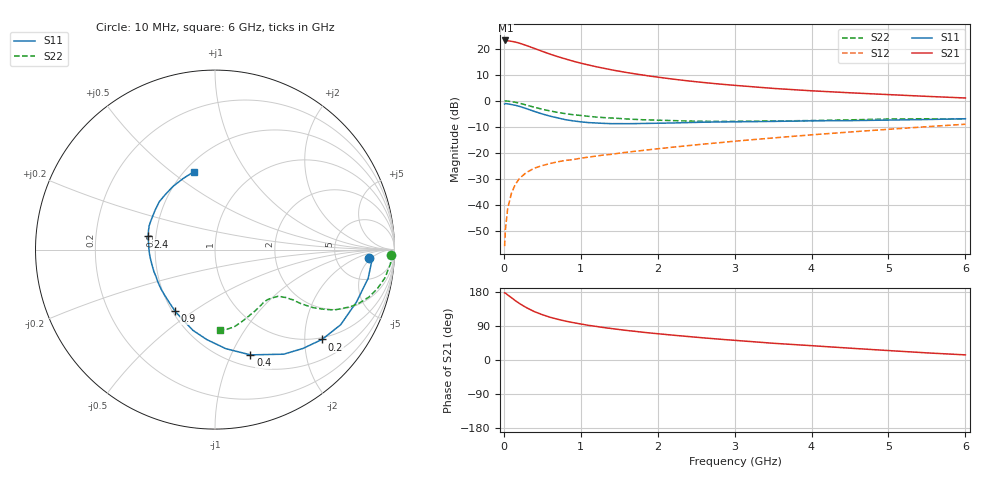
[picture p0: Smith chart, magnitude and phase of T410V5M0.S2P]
! Infineon Technologies  Discrete & RF Semiconductors
! BFR182T
! Si NPN RF Bipolar Junction Transistor in SC75
! VCE = 10 V  IC = 5 mA
! Common Emitter S-Parameters:  October  1999
# GHz  S  MA  R  50
!  f  S11  S21  S12  S22
! GHz  MAG  ANG  MAG  ANG  MAG  ANG  MAG  ANG
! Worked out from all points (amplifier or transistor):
!   36 points, 10 MHz to 6 GHz, reference 50 ohm
!   highest |S21| = 23.1 dB at 20 MHz (marker M1)
!   |S21| within 3 dB of that: start of sweep to 391.5 MHz
!   unconditionally stable (mu >= 1): 1.532 GHz to 4.23 GHz
!   at 250 MHz: K = 0.27, MSG = 25.1 dB, |S12| = -28.7 dB
!   at 1.4 GHz: K = 0.98, MSG = 16.2 dB, |S12| = -20.6 dB
!   at 6 GHz: K = 0.86, MSG = 5.0 dB, |S12| = -9.1 dB
!   S11 on the Smith chart (normalised r, x): 10 MHz: 12, -4; 200 MHz: 0.95, -2.42; 400 MHz: 0.62, -1.19; 900 MHz: 0.52, -0.43; 2.4 GHz: 0.45, +0.08; 6 GHz: 0.55, +0.60
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0.01  0.8613 -3.2  14.28 177.1  0.0016 81.4  0.9803 -1.7
0.02  0.8788 -2.9  14.34 176.6  0.0033 83.2  0.9873 -1.9
0.05  0.8682 -10.6  14.16 171.7  0.0085 82.9  0.9799 -4.8
0.1  0.8407 -20.3  13.79 164.3  0.0169 80.2  0.9601 -9.4
0.15  0.8157 -30.9  13.36 156.5  0.0247 74.6  0.9301 -13.6
0.2  0.7786 -40.0  12.77 149.6  0.0315 71.8  0.8966 -17.2
0.25  0.7373 -48.3  12.06 143.3  0.0369 66.2  0.8565 -20.4
0.3  0.6972 -56.7  11.38 137.5  0.0422 64.2  0.8189 -22.9
0.4  0.6188 -71.4  10.04 127.4  0.0507 59.0  0.7441 -26.9
0.5  0.5551 -83.8  8.857 119.6  0.0566 55.5  0.6843 -29.0
0.6  0.5038 -95.1  7.836 112.9  0.0619 53.7  0.6353 -30.6
0.7  0.4663 -105.3  7.019 107.5  0.0668 53.5  0.5943 -31.5
0.9  0.4089 -123.0  5.74 98.7  0.0737 52.9  0.536 -32.6
1.1  0.3786 -137.8  4.848 91.5  0.0823 53.5  0.5001 -33.4
1.3  0.3659 -150.3  4.19 85.6  0.0904 54.2  0.4722 -34.3
1.6  0.3611 -165.8  3.464 77.9  0.1022 55.8  0.4446 -35.9
2.2  0.3724 174.1  2.591 65.5  0.1278 58.4  0.4136 -41.0
2.4  0.3794 168.9  2.392 61.9  0.137 59.1  0.4059 -43.1
3.5  0.3991 147.0  1.72 44.2  0.192 59.4  0.4071 -55.9
4.5  0.4134 131.9  1.416 31.2  0.2499 57.2  0.4277 -69.3
5.5  0.4341 114.1  1.209 18.8  0.3161 53.4  0.4488 -81.4
6  0.4492 105.4  1.125 13.5  0.3523 50.4  0.4488 -86.4
